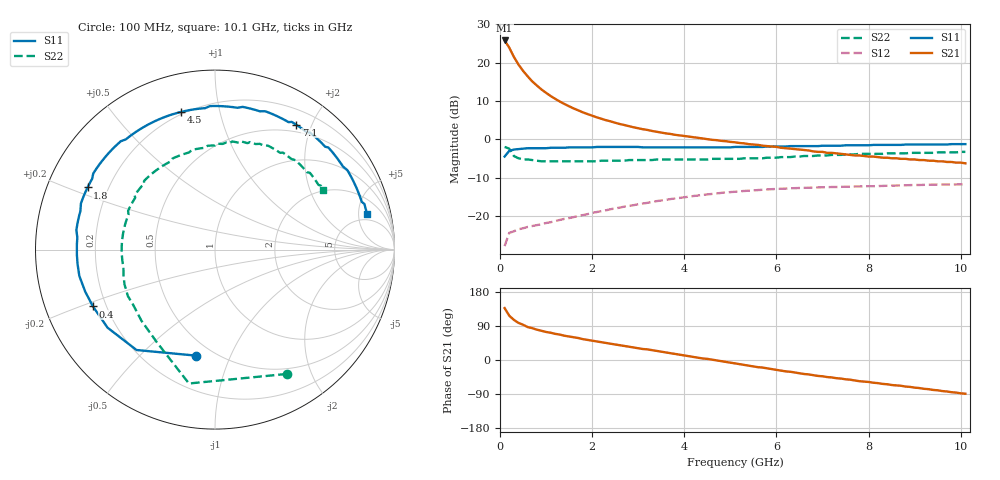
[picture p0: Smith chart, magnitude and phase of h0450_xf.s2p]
!HBFP-0450
!S and NOISE PARAMETERS at Vce=0.5V  Ic=20mA.  LAST UPDATED  09-04-98
# GHZ S MA R  50
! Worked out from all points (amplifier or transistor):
!   101 points, 100 MHz to 10.1 GHz, reference 50 ohm
!   highest |S21| = 25.8 dB at 100 MHz (marker M1)
!   |S21| within 3 dB of that: start of sweep to 248.2 MHz
!   unconditionally stable (mu >= 1): 2.419 GHz to end of sweep
!   at 1.7 GHz: K = 0.90, MSG = 13.7 dB, |S12| = -19.9 dB
!   at 5.1 GHz: K = 1.11, MAG = 4.4 dB, |S12| = -13.6 dB
!   at 10.1 GHz: K = 1.10, MAG = 0.8 dB, |S12| = -11.7 dB
!   lowest NFmin = 1.29 dB at 1.8 GHz
!   S11 on the Smith chart (normalised r, x): 100 MHz: 0.41, -0.75; 400 MHz: 0.15, -0.22; 1.8 GHz: 0.12, +0.23; 4.5 GHz: 0.19, +0.76; 7.1 GHz: 0.40, +1.77; 10.1 GHz: 3.95, +6.36
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0.1  0.6 -100.0  19.39 137.0  0.041 54.0  0.8 -60.0
0.2  0.71 -128.0  15.68 117.0  0.061 40.0  0.76 -101.0
0.3  0.74 -144.0  11.9 106.0  0.064 30.0  0.61 -122.0
0.4  0.75 -155.0  9.44 98.0  0.068 27.0  0.57 -136.0
0.5  0.76 -162.0  7.81 93.0  0.07 25.0  0.55 -146.0
0.6  0.77 -169.0  6.63 87.0  0.073 24.0  0.55 -152.0
0.7  0.77 -174.0  5.69 84.0  0.075 24.0  0.54 -159.0
0.8  0.77 -178.0  5.03 80.0  0.077 24.0  0.53 -164.0
0.9  0.77 178.0  4.47 77.0  0.079 25.0  0.52 -169.0
1.1  0.78 172.0  3.67 72.0  0.084 25.0  0.52 -177.0
1.3  0.78 166.0  3.11 67.0  0.09 26.0  0.52 177.0
1.5  0.79 161.0  2.7 62.0  0.095 26.0  0.52 171.0
1.8  0.79 154.0  2.25 55.0  0.104 26.0  0.52 164.0
2.1  0.8 148.0  1.94 49.0  0.114 25.0  0.52 158.0
2.6  0.8 138.0  1.59 39.0  0.13 22.0  0.53 149.0
3.5  0.79 122.0  1.23 22.0  0.161 15.0  0.55 134.0
4.5  0.79 104.0  1.01 3.0  0.193 3.0  0.55 117.0
5.1  0.8 92.0  0.92 -9.0  0.209 -6.0  0.56 106.0
6.8  0.82 62.0  0.7 -40.0  0.237 -30.0  0.61 77.0
7.1  0.83 57.0  0.67 -45.0  0.24 -34.0  0.62 73.0
8.5  0.85 36.0  0.57 -66.0  0.251 -52.0  0.66 54.0
10.1  0.87 13.0  0.49 -89.0  0.261 -75.0  0.69 29.0
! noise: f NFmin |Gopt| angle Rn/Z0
1.8  1.29  0.56  -165  0.05
2  1.35  0.58  -162  0.05
2.5  1.46  0.59  -150  0.09
3.5  1.72  0.65  -131  0.2
4  1.87  0.66  -120  0.33
5  2.12  0.69  -100  0.62
5.5  2.26  0.72  -89  0.88
7  2.63  0.76  -61  1.82
8  2.89  0.77  -45  2.47
10  3.4  0.8  -16  3.99
